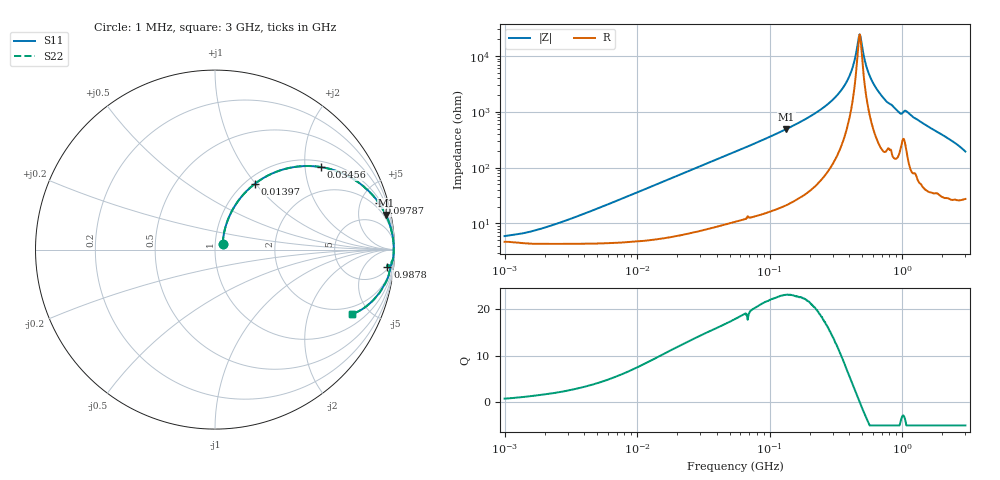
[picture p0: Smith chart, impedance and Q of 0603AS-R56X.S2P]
!s-Parameter Generated by FASTRON Sdn. Bhd.
!FASTRON P/N : 0603AS-R56X
!Keysight Technologies: E4991B_MY54100416_A.01.15
!Date created: Tue Oct 17 15:13:57 2023
!Version  : Rev01 Tue Oct 17 15:13:57 2023
!Data & Calibration Information:
!Freq	S11	S21	S12	S22
!PortZ  Port1:50+j0  Port2:50+j0
!When reading reference impedance value at option line is always used.
! Remarks : This data is being provided solely for informational purposes.
# Hz S dB R 50
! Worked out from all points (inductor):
!   1601 points, 1 MHz to 3 GHz, reference 50 ohm
!   read as one part in series: L = 571 nH near 3.618 MHz
!   highest Q = 23.1 at 133.5 MHz (marker M1), where L = 585 nH
!   self-resonance near 475.8 MHz
!   S11 on the Smith chart (normalised r, x): 1 MHz: 1.09, +0.07; 13.97 MHz: 1.10, +0.99; 34.56 MHz: 1.16, +2.43; 97.87 MHz: 1.32, +6.96; 987.8 MHz: 6, -18; 3 GHz: 1.55, -3.85
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1000000  -24.92 35.7  -0.40 -2.0  -0.40 -2.0  -24.92 35.7
3804036  -17.31 65.0  -0.44 -7.5  -0.44 -7.5  -17.31 65.0
1.397259e7  -7.34 58.7  -1.32 -25.3  -1.32 -25.3  -7.34 58.7
1.447069e7  -7.10 58.1  -1.38 -26.1  -1.38 -26.1  -7.10 58.1
3.456417e7  -2.51 37.9  -4.22 -48.3  -4.22 -48.3  -2.51 37.9
5.477226e7  -1.24 26.8  -6.90 -60.0  -6.90 -60.0  -1.24 26.8
9.787053e7  -0.45 15.8  -11.29 -71.6  -11.29 -71.6  -0.45 15.8
1.334721e8  -0.25 11.4  -14.07 -76.1  -14.07 -76.1  -0.25 11.4
2.083556e8  -0.10 6.5  -18.86 -80.7  -18.86 -80.7  -0.10 6.5
2.913464e8  -0.06 3.7  -23.87 -82.4  -23.87 -82.4  -0.06 3.7
3.649251e8  -0.04 2.0  -29.28 -81.3  -29.28 -81.3  -0.04 2.0
4.177151e8  -0.04 1.0  -35.18 -75.7  -35.18 -75.7  -0.04 1.0
4.639993e8  -0.04 0.2  -45.08 -42.3  -45.08 -42.3  -0.04 0.2
4.781416e8  -0.04 -0.0  -47.76 0.1  -47.76 0.1  -0.04 -0.0
4.92715e8  -0.04 -0.2  -45.01 42.2  -45.01 42.2  -0.04 -0.2
5.364635e8  -0.04 -0.8  -36.36 72.8  -36.36 72.8  -0.04 -0.8
5.81181e8  -0.04 -1.4  -31.93 78.4  -31.93 78.4  -0.04 -1.4
7.925923e8  -0.11 -3.9  -23.24 77.3  -23.24 77.3  -0.11 -3.9
9.878038e8  -0.30 -5.8  -19.62 68.1  -19.62 68.1  -0.30 -5.8
1.075512e9  -0.20 -5.3  -20.44 73.3  -20.44 73.3  -0.20 -5.3
1.980367e9  -0.42 -13.9  -12.38 71.8  -12.38 71.8  -0.42 -13.9
3e9  -1.49 -25.4  -7.27 56.5  -7.27 56.5  -1.49 -25.4
